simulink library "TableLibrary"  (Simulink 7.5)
settings: Solver=ode45  StartTime=0.0  StopTime=10.0  RelTol=1e-3

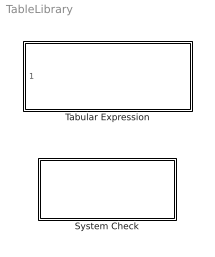
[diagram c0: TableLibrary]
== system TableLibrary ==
  System Check : Subsystem
  Tabular Expression : Subsystem

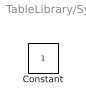
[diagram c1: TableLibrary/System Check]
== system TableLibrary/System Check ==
  Constant : Constant  OutDataType=fixdt(1, 16)  OutScaling=2^0

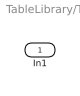
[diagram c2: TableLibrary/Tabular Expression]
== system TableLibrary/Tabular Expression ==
  In1 : Inport  OutDataType=fixdt(1, 16)  OutScaling=2^0
